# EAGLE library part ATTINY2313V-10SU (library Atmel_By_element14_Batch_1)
Microcontroller with 2K Bytes In-System Programmable Flash
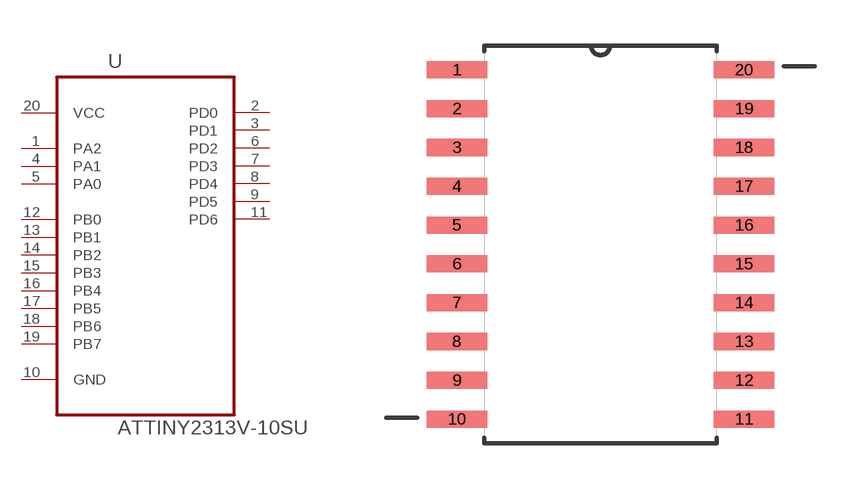
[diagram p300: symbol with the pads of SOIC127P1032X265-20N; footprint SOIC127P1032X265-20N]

Designator prefix U

## ATTINY2313V-10SU (MPN: ATTINY2313V-10SU; OC_FARNELL: 9171622; OC_NEWARK: 01M6917; PACKAGE: SOIC-16; SUPPLIER: Atmel)  [SOIC127P1032X265-20N]
1  PA2
2  PD0
3  PD1
4  PA1
5  PA0
6  PD2
7  PD3
8  PD4
9  PD5
10  GND  pas
11  PD6
12  PB0
13  PB1
14  PB2
15  PB3
16  PB4
17  PB5
18  PB6
19  PB7
20  VCC  pwr

## Footprint SOIC127P1032X265-20N (pad centres in mm)
smd 1.981 x 0.559: 1 -4.699,5.715; 2 -4.699,4.445; 3 -4.699,3.175; 4 -4.699,1.905; 5 -4.699,0.635; 6 -4.699,-0.635; 7 -4.699,-1.905; 8 -4.699,-3.175; 9 -4.699,-4.445; 10 -4.699,-5.715; 11 4.699,-5.715; 12 4.699,-4.445; 13 4.699,-3.175; 14 4.699,-1.905; 15 4.699,-0.635; 16 4.699,0.635; 17 4.699,1.905; 18 4.699,3.175; 19 4.699,4.445; 20 4.699,5.715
